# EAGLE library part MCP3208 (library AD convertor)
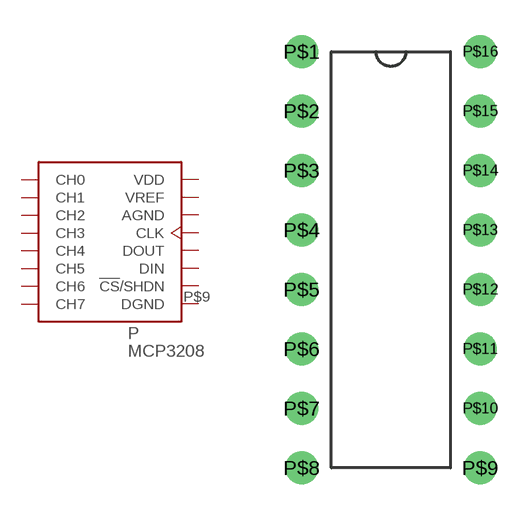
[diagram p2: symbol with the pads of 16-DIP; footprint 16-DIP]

Designator prefix P

## MCP3208DIP  [16-DIP]
P$1  CH0  in
P$2  CH1  in
P$3  CH2  in
P$4  CH3  in
P$5  CH4  in
P$6  CH5  in
P$7  CH6  in
P$8  CH7  in
P$9  DGND  pwr
P$10  !CS!/SHDN  sup
P$11  DIN  in
P$12  DOUT  out
P$13  CLK  in
P$14  AGND  pwr
P$15  VREF  pwr
P$16  VDD  pwr

## Footprint 16-DIP (pad centres in mm)
drill 0.9: P$1 -5.08,10.16; P$2 -5.08,7.62; P$3 -5.08,5.08; P$4 -5.08,2.54; P$5 -5.08,0; P$6 -5.08,-2.54; P$7 -5.08,-5.08; P$8 -5.08,-7.62; P$9 2.54,-7.62; P$10 2.54,-5.08; P$11 2.54,-2.54; P$12 2.54,0; P$13 2.54,2.54; P$14 2.54,5.08; P$15 2.54,7.62; P$16 2.54,10.16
